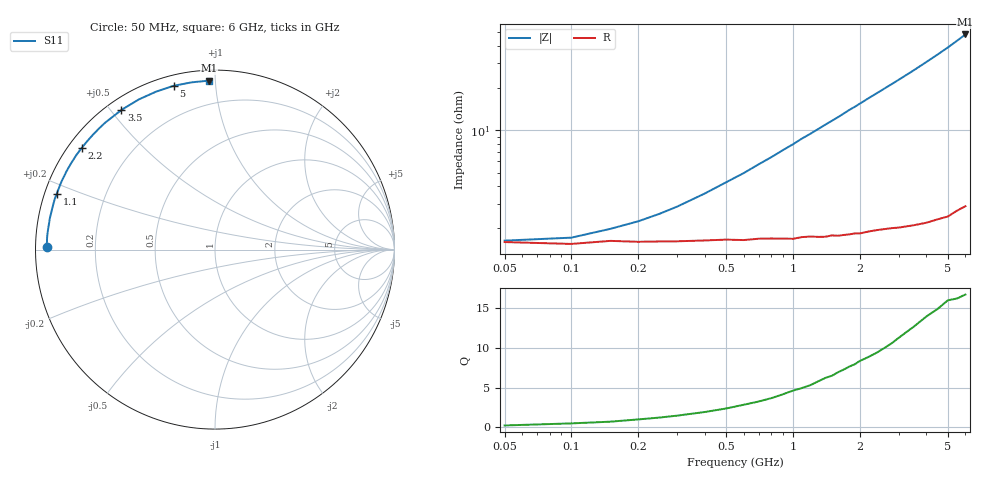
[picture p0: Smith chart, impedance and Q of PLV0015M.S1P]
! Infineon Technologies  Discrete & RF Semiconductors
! BAR 64-04W /-05W /-06W
! Si PIN Diode in SOT323
! IF = 15 mA
! S-Parameters:  October  2008
# GHz  S  MA  R  50
!  f  S11
! GHz  MAG  ANG
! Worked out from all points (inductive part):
!   34 points, 50 MHz to 6 GHz, reference 50 ohm
!   read as one part to ground: L = 1.24 nH near 700 MHz
!   highest Q = 16.8 at 6 GHz (marker M1), where L = 1.28 nH
!   S11 on the Smith chart (normalised r, x): 50 MHz: 0.03, +0.01; 1.1 GHz: 0.03, +0.17; 2.2 GHz: 0.04, +0.34; 3.5 GHz: 0.04, +0.53; 5 GHz: 0.05, +0.78; 6 GHz: 0.06, +0.96
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0.05  0.9381 179.2
0.1  0.9399 178.3
0.15  0.9369 177.4
0.2  0.9379 176.4
0.4  0.9367 172.8
0.5  0.936 171.0
0.6  0.9366 169.3
0.7  0.9355 167.5
0.8  0.9354 165.8
0.9  0.9358 164.0
1  0.9363 162.3
1.1  0.9348 160.5
1.2  0.9346 158.9
1.3  0.9353 157.2
1.4  0.9356 155.5
1.6  0.9354 152.3
1.8  0.9349 148.9
2  0.935 145.8
2.2  0.934 142.6
2.4  0.9337 139.6
2.6  0.9339 136.6
3  0.9352 130.8
3.5  0.9366 123.8
4  0.9382 116.9
4.5  0.9393 110.4
5  0.9413 104.1
5.5  0.9409 97.9
6  0.9421 92.0
